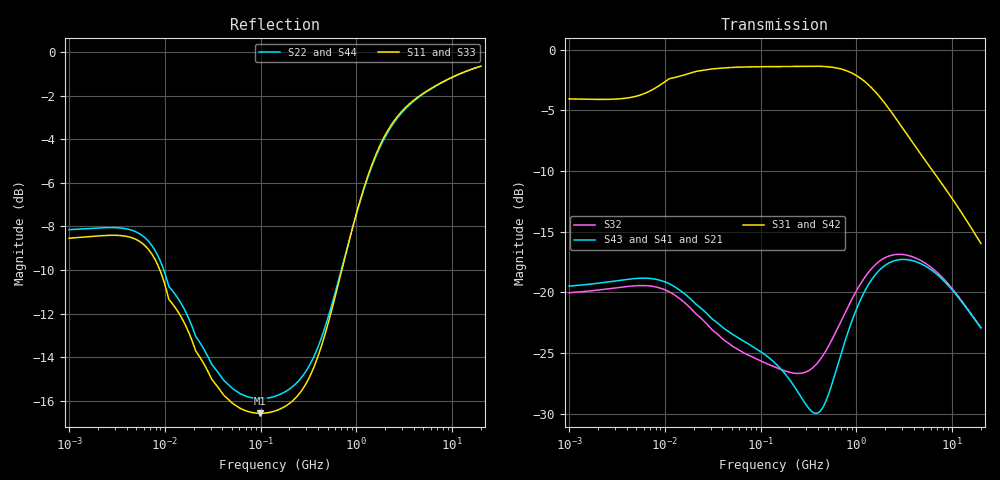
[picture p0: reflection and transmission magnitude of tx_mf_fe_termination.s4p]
! Created Wed Jul 29 12:28:18 2015
# hz S db R 50
! 4 Port Network Data from SP1.SP block
! freq  dbS11  angS11  dbS12  angS12  dbS13  angS13  dbS14  angS14
!  dbS21  angS21  dbS22  angS22  dbS23  angS23  dbS24  angS24
!  dbS31  angS31  dbS32  angS32  dbS33  angS33  dbS34  angS34
!  dbS41  angS41  dbS42  angS42  dbS43  angS43  dbS44  angS44
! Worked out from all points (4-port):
!   861 points, 1 MHz to 20 GHz, reference 50 ohm
!   strongest paths, dB at 1 MHz, 11.89 MHz, 141.4 MHz, 1.682 GHz, 20 GHz:
!     S31: -4.0, -2.3, -1.4, -3.7, -16.0
!     S42: -4.3, -2.5, -1.5, -3.8, -16.0
!     S43: -19.5, -19.4, -25.8, -18.3, -22.9
!     S41: -19.5, -19.4, -25.8, -18.3, -22.9
!     S21: -19.5, -19.4, -25.8, -18.3, -22.9
!     S32: -20.0, -20.1, -26.2, -17.5, -22.9
!   lowest |S11| = -16.6 dB at 98.96 MHz (marker M1), VSWR 1.35, Z = 37.1 - j0.638 ohm
!   |S11| at or under -10 dB: 8.868 MHz to 705.5 MHz (696.7 MHz wide, 195 % of centre)
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1000000  -8.54 176.3  -20.03 -0.2  -4.05 2.2  -20.03 -0.2
         -19.48 0.2  -8.15 176.5  -19.48 0.2  -4.30 2.2
         -4.05 2.2  -20.03 -0.2  -8.54 176.3  -20.03 -0.2
         -19.48 0.2  -4.30 2.2  -19.48 0.2  -8.15 176.5
9445687  -10.33 157.8  -19.72 -18.4  -2.77 9.1  -19.72 -18.4
         -19.07 -16.0  -9.84 158.8  -19.07 -16.0  -2.98 9.4
         -2.77 9.1  -19.72 -18.4  -10.33 157.8  -19.72 -18.4
         -19.07 -16.0  -2.98 9.4  -19.07 -16.0  -9.84 158.8
9.896414e7  -16.58 -176.7  -25.64 -57.1  -1.39 -0.6  -25.64 -57.1
            -24.86 -44.7  -15.91 -177.4  -24.86 -44.7  -1.51 -0.5
            -1.39 -0.6  -25.64 -57.1  -16.58 -176.7  -25.64 -57.1
            -24.86 -44.7  -1.51 -0.5  -24.86 -44.7  -15.91 -177.4
4.032961e8  -13.89 -139.8  -25.72 -164.6  -1.35 -8.8  -25.72 -164.6
            -29.91 -155.1  -13.47 -142.9  -29.91 -155.1  -1.51 -8.8
            -1.35 -8.8  -25.72 -164.6  -13.89 -139.8  -25.72 -164.6
            -29.91 -155.1  -1.51 -8.8  -29.91 -155.1  -13.47 -142.9
1.176889e9  -6.36 -134.1  -18.97 87.4  -2.50 -27.4  -18.97 87.4
            -20.17 79.0  -6.42 -135.8  -20.17 79.0  -2.65 -26.9
            -2.50 -27.4  -18.97 87.4  -6.36 -134.1  -18.97 87.4
            -20.17 79.0  -2.65 -26.9  -20.17 79.0  -6.42 -135.8
2.487787e9  -3.15 -149.6  -16.89 32.4  -5.46 -41.4  -16.89 32.4
            -17.40 28.8  -3.23 -150.0  -17.40 28.8  -5.51 -40.6
            -5.46 -41.4  -16.89 32.4  -3.15 -149.6  -16.89 32.4
            -17.40 28.8  -5.51 -40.6  -17.40 28.8  -3.23 -150.0
2e10  -0.65 -171.6  -22.91 -41.8  -15.97 -59.0  -22.91 -41.8
      -22.94 -41.7  -0.65 -171.5  -22.94 -41.7  -15.96 -59.0
      -15.97 -59.0  -22.91 -41.8  -0.65 -171.6  -22.91 -41.8
      -22.94 -41.7  -15.96 -59.0  -22.94 -41.7  -0.65 -171.5
